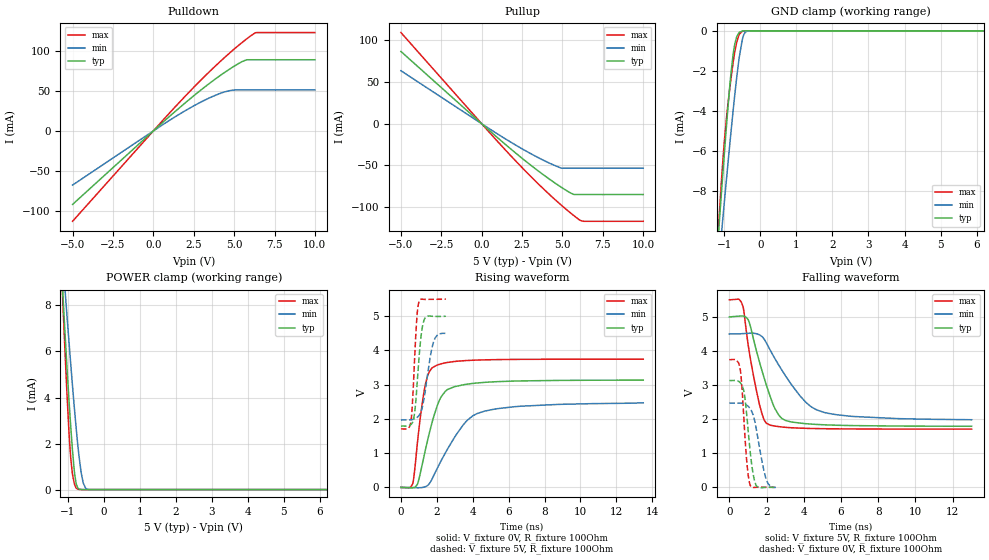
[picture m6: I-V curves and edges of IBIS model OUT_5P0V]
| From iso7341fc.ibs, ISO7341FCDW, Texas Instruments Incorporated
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|   OUT_5P0V Model
[Model]   OUT_5P0V
Model_type   3-state
Polarity   Non-Inverting
Vmeas = 2.5
Vref = 0
Cref = 15pF
Rref = 150
|   typ   min   max
|   (nom PVT)   (fast PVT)   (slow PVT)
C_comp   4.042e-13   2.684e-13   4.460e-13
| Where   Nom PVT is  Nominal Process, 5.0V, 27C
|   Fast PVT is Strong Process, 5.5V, -40C
|   Slow PVT is Weak Process, 4.5V, 150C
[Voltage Range]   5   4.5   5.5
[Temperature Range]   27   150   -40
[Pullup Reference]   5   4.5   5.5
[Pulldown Reference]   0   0   0
[Power Clamp Reference]   5   4.5   5.5
[GND Clamp Reference]   0   0   0
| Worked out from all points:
|   slope of the pulldown table from 0 to 0.75 V, typ, clamps not added: 54.8 ohm
|   slope of the pullup table from 0 to 0.75 V, typ, clamps not added: 58.4 ohm
|   GND clamp passes 1 mA (typ) near -0.74 V on its own axis
|   POWER clamp passes 1 mA (typ) near -0.83 V on its own axis
|   falling waveform, V_fixture 5V, R_fixture 100Ohm: 20-80 % time 1.06ns typ, 1.91ns min, 728ps max; typ from 5 V to 1.79 V
|   rising waveform, V_fixture 0V, R_fixture 100Ohm: 20-80 % time 946ps typ, 1.77ns min, 546ps max; typ from 0 V to 3.13 V
|   rising waveform, V_fixture 5V, R_fixture 100Ohm: 20-80 % time 294ps typ, 454ps min, 219ps max; typ from 1.79 V to 5 V
|   falling waveform, V_fixture 0V, R_fixture 100Ohm: 20-80 % time 350ps typ, 507ps min, 270ps max; typ from 3.13 V to 0 V
[Pulldown]
|   Voltage   I(typ)   I(min)   I(max)
-5V       -92.05mA   -67.84mA   -113.2mA
577mV     10.56mA    7.757mA    13.02mA
2.497V    43.95mA    31.35mA    54.51mA
3.553V    60.75mA    42.14mA    75.77mA
4.418V    73.37mA    48.92mA    92.14mA
4.999V    81.05mA    51.31mA    102.5mA
5.78V     89.18mA    51.32mA    115.4mA
6.335V    89.18mA    51.32mA    123.1mA
10V       89.18mA    51.32mA    123.2mA
[GND Clamp]
|   Voltage   I(typ)   I(min)   I(max)
-5V       -110.2mA   -89.81mA   -133.4mA
-1.167V   -10.19mA   -11.81mA   -9.891mA
-1.143V   -9.614mA   -11.35mA   -9.218mA
-1.056V   -7.455mA   -9.63mA    -6.826mA
-941mV    -4.71mA    -7.385mA   -4.33mA
-845mV    -2.647mA   -5.57mA    -2.788mA
-760mV    -1.21mA    -4.027mA   -1.611mA
-655mV    -285.7uA   -2.274mA   -550uA
-500mV    -9.741uA   -414.6uA   -17.95uA
-423.5mV  -1.198uA   -82.08uA   -1.482uA
-290mV    -19.17nA   -2.467uA   0A
10V       0A         0A         0A
[Pullup]
|   Voltage   I(typ)   I(min)   I(max)
-5V       86.63mA    63.54mA    109.3mA
700mV     -12mA      -8.815mA   -15.19mA
2.832V    -46.56mA   -33.69mA   -59.17mA
4.036V    -64.25mA   -45.78mA   -81.96mA
4.894V    -75.71mA   -52.92mA   -97.03mA
5.505V    -83.08mA   -53.29mA   -107mA
5.72V     -84.8mA    -53.29mA   -110.4mA
5.89V     -84.82mA   -53.29mA   -112.9mA
6.077V    -84.82mA   -53.29mA   -115.6mA
6.322V    -84.82mA   -53.29mA   -116.9mA
10V       -84.82mA   -53.29mA   -116.9mA
[POWER Clamp]
|   Voltage   I(typ)   I(min)   I(max)
-5V       131.5mA    105.6mA    159.1mA
-1.293V   13.33mA    13.59mA    14.08mA
-1.13V    8.417mA    9.9mA      7.997mA
-1.089V   7.25mA     9.031mA    6.551mA
-1.036V   5.752mA    7.899mA    4.703mA
-963mV    3.883mA    6.422mA    2.5mA
-913.5mV  2.715mA    5.439mA    1.356mA
-805mV    678.4uA    3.391mA    212.5uA
-720mV    74.85uA    1.965mA    18.11uA
-567.5mV  735.3nA    284.1uA    116.9nA
-414.5mV  0A         6.65uA     0A
10V       0A         0A         0A
[Ramp]
R_load = 100
|   typ   min   max
dV/dt_r   1.88108/9.42646e-10   1.48307/1.76837e-09   2.24802/5.46847e-10
dV/dt_f   1.92542/1.05591e-09   1.5171/1.92217e-09   2.27514/7.2543e-10
[Falling Waveform]
V_fixture = 5V
V_fixture_min = 4.5V
V_fixture_max = 5.5V
R_fixture = 100Ohm
|   Time   V(typ)   V(min)   V(max)
0s        5V         4.5V       5.5V
720ps     5.027V     4.51V      5.329V
1.022ns   4.908V     4.52V      4.147V
1.392ns   4.145V     4.515V     3.017V
1.75ns    3.432V     4.427V     2.17V
2.006ns   2.976V     4.223V     1.877V
2.456ns   2.306V     3.771V     1.798V
2.828ns   2.02V      3.435V     1.771V
4.696ns   1.846V     2.272V     1.725V
13.02ns   1.793V     1.984V     1.708V
[Rising Waveform]
V_fixture = 0V
V_fixture_min = 0V
V_fixture_max = 0V
R_fixture = 100Ohm
|   Time   V(typ)   V(min)   V(max)
0s        717.1pV    3.009nV    690.4pV
664ps     -10.66mV   -5.881mV   120.6mV
924ps     99.11mV    -9.583mV   1.332V
1.324ns   1.004V     13.2mV     2.902V
1.526ns   1.467V     76.73mV    3.317V
1.842ns   2.095V     364mV      3.526V
2.578ns   2.853V     1.105V     3.648V
3.464ns   2.996V     1.823V     3.7V
4.252ns   3.051V     2.159V     3.72V
13.5ns    3.135V     2.472V     3.747V
[Rising Waveform]
V_fixture = 5V
V_fixture_min = 4.5V
V_fixture_max = 5.5V
R_fixture = 100Ohm
|   Time   V(typ)   V(min)   V(max)
0s        1.793V     1.97V      1.71V
562ps     1.84V      1.976V     1.959V
640ps     1.893V     1.983V     2.459V
786ps     2.29V      2.008V     4.019V
906ps     3.065V     2.047V     5.083V
1.02ns    3.876V     2.111V     5.446V
1.15ns    4.54V      2.259V     5.497V
1.292ns   4.896V     2.615V     5.493V
1.822ns   4.997V     4.263V     5.495V
2.5ns     5V         4.5V       5.5V
[Falling Waveform]
V_fixture = 0V
V_fixture_min = 0V
V_fixture_max = 0V
R_fixture = 100Ohm
|   Time   V(typ)   V(min)   V(max)
0s        3.134V     2.472V     3.745V
582ps     3.073V     2.471V     3.483V
682ps     2.992V     2.465V     2.912V
824ps     2.685V     2.443V     1.624V
962ps     1.977V     2.4V       619.6mV
1.12ns    1.058V     2.311V     64.08mV
1.29ns    360mV      2.111V     -3.958mV
1.49ns    18.99mV    1.584V     2.567mV
1.956ns   700uV      283.5mV    2.491mV
2.5ns     3.135uV    17.33uV    541.4nV
